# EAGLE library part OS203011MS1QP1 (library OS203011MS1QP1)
Slide Switches DP3T On-On-On Source: Datasheet
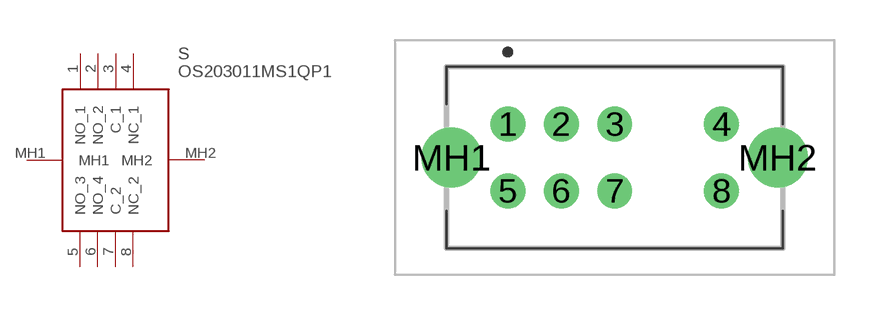
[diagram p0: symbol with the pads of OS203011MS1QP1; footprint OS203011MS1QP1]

Designator prefix S

## OS203011MS1QP1 (Arrow_Part_Number: OS203011MS1QP1; Arrow_Price-Stock: https://www.arrow.com/en/products/os203011ms1qp1/ck?region=nac; Description: Slide Switches DP3T On-On-On; Height: 8mm; Manufacturer_Name: C & K COMPONENTS; Manufacturer_Part_Number: OS203011MS1QP1; Mouser_Part_Number: 611-OS203011MS1QP1; Mouser_Price-Stock: https://www.mouser.co.uk/ProductDetail/CK/OS203011MS1QP1?qs=vOb5o%2F429vPBgVy%2FFFX7mQ%3D%3D)  [OS203011MS1QP1]
1  NO_1
2  NO_2
3  C_1
4  NC_1
5  NO_3
6  NO_4
7  C_2
8  NC_2
MH1  MH1
MH2  MH2

## Footprint OS203011MS1QP1 (pad centres in mm)
OS203011MS1QP1-2
drill 0.8 pad 1.3: 1 0,0; 2 2,0; 3 4,0; 4 8,0; 5 0,-2.5; 6 2,-2.5; 7 4,-2.5; 8 8,-2.5
drill 1.5 pad 2.25: MH1 -2.1,-1.25; MH2 10.1,-1.25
